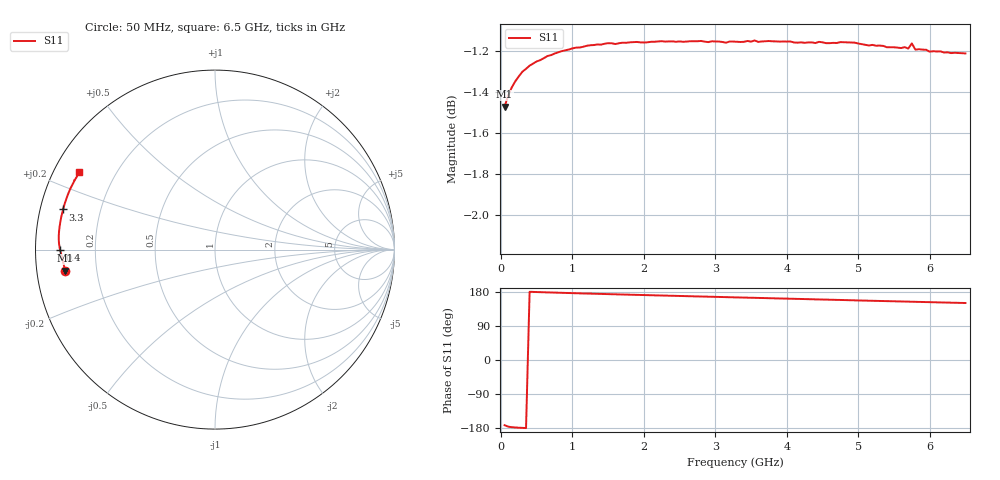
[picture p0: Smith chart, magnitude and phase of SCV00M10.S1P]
! Infineon Technologies  Discrete & RF Semiconductors
! BAR63-02L
! Si PIN Diode in TSLP-2
! IF = 0.1 mA
! S-Parameters:  March  2002
# GHz  S  MA  R  50
!  f  S11
! GHz  MAG  ANG
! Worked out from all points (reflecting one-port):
!   130 points, 50 MHz to 6.5 GHz, reference 50 ohm
!   lowest |S11| = -1.5 dB at 50 MHz (marker M1), VSWR 11.84, Z = 4.24 - j3.47 ohm
!   phase of S11 starts at -172 deg and turns -38 deg over the sweep
!   S11 on the Smith chart (normalised r, x): 50 MHz: 0.08, -0.07; 400 MHz: 0.07, +0.00; 3.3 GHz: 0.07, +0.13; 6.5 GHz: 0.07, +0.26
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0.05  0.8442 -172.0
0.1  0.8495 -175.9
0.15  0.8533 -177.3
0.2  0.8563 -178.1
0.25  0.8587 -178.7
0.4  0.8638 180.0
0.45  0.8648 179.6
0.85  0.8708 177.2
0.9  0.8712 177.0
1.15  0.873 175.6
1.5  0.8747 173.9
1.7  0.875 172.8
1.8  0.8751 172.4
2.15  0.8754 170.6
2.5  0.8756 169.0
2.8  0.8758 167.5
3.3  0.8754 165.2
3.75  0.8758 163.1
4.1  0.8751 161.4
4.25  0.8749 160.8
4.4  0.8748 160.0
4.9  0.875 157.7
5.05  0.8742 156.9
5.7  0.8721 154.0
5.75  0.8746 153.8
5.8  0.8716 153.5
6.1  0.8707 152.1
6.5  0.8697 150.4
